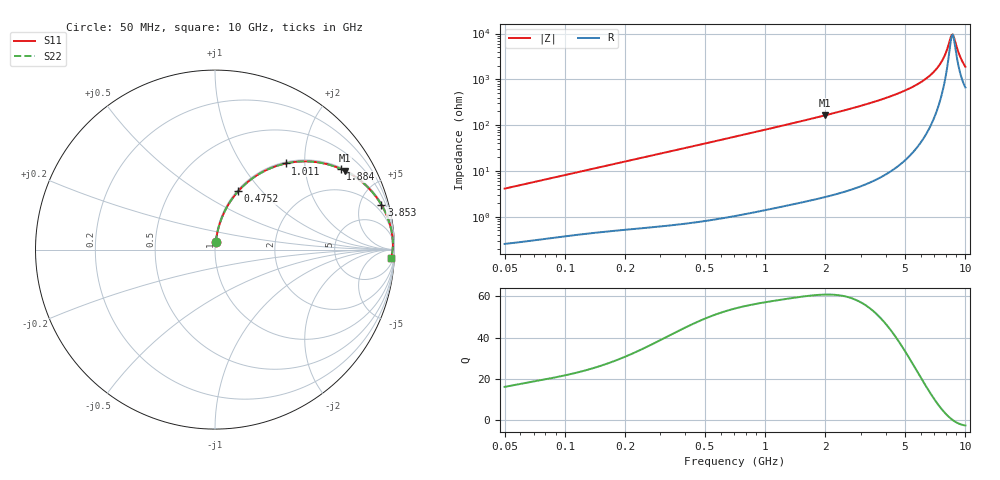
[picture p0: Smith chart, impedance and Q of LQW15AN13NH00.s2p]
!Murata Part Number: LQW15AN13NH00
!These Parameters are Measured in Series Mode Connection
!  o--[Z]--o
!Port1  Port2
!  o-------o
!Freq. Start=50[MHz] Stop=10[GHz], 401[Steps]
# Hz S RI R 50
!Freq.(Hz)	S 11(Real)	S 11(Imag)	S 21(Real)	S 21(Imag)	S 12(Real)	S 12(Imag)	S 22(Real)	S 22(Imag)
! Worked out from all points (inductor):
!   401 points, 50 MHz to 10 GHz, reference 50 ohm
!   read as one part in series: L = 13 nH near 51.34 MHz
!   highest Q = 60.9 at 1.987 GHz (marker M1), where L = 13 nH
!   self-resonance near 8.53 GHz
!   S11 on the Smith chart (normalised r, x): 50 MHz: 1.01, +0.08; 475.2 MHz: 1.02, +0.75; 1.011 GHz: 1.03, +1.60; 1.884 GHz: 1.05, +3.07; 3.853 GHz: 1.15, +7.37; 10 GHz: 14, -35
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5e7  0.00419 0.0406  0.9958 -0.0406  0.9958 -0.0406  0.00419 0.0406
1.214486e8  0.0134 0.0958  0.9866 -0.0958  0.9866 -0.0958  0.0134 0.0958
2.949953e8  0.0569 0.219  0.9431 -0.219  0.9431 -0.219  0.0569 0.219
4.752343e8  0.1287 0.3247  0.8713 -0.3247  0.8713 -0.3247  0.1287 0.3247
7.071068e8  0.2422 0.4193  0.7578 -0.4193  0.7578 -0.4193  0.2422 0.4193
1.011124e9  0.3935 0.4799  0.6065 -0.4799  0.6065 -0.4799  0.3935 0.4799
1.717543e9  0.6568 0.4666  0.3432 -0.4666  0.3432 -0.4666  0.6568 0.4666
1.884411e9  0.6996 0.4503  0.3004 -0.4503  0.3004 -0.4503  0.6996 0.4503
1.986945e9  0.7229 0.4394  0.2771 -0.4394  0.2771 -0.4394  0.7229 0.4394
2.766943e9  0.8458 0.3527  0.1542 -0.3527  0.1542 -0.3527  0.8458 0.3527
3.853138e9  0.927 0.2501  0.073 -0.2501  0.073 -0.2501  0.927 0.2501
4.171863e9  0.9408 0.225  0.0592 -0.225  0.0592 -0.225  0.9408 0.225
5.583245e9  0.9761 0.1344  0.0239 -0.1344  0.0239 -0.1344  0.9761 0.1344
6.810442e9  0.9882 0.0736  0.0118 -0.0736  0.0118 -0.0736  0.9882 0.0736
7.276762e9  0.9902 0.0534  0.00984 -0.0534  0.00984 -0.0534  0.9902 0.0534
7.672705e9  0.9909 0.037  0.00906 -0.037  0.00906 -0.037  0.9909 0.037
7.983737e9  0.991 0.0247  0.00899 -0.0247  0.00899 -0.0247  0.991 0.0247
8.418147e9  0.9903 0.00803  0.00967 -0.00803  0.00967 -0.00803  0.9903 0.00803
8.530394e9  0.99 0.00383  0.00999 -0.00383  0.00999 -0.00383  0.99 0.00383
8.759398e9  0.9892 -0.00462  0.0108 0.00462  0.0108 0.00462  0.9892 -0.00462
9.48396e9  0.9846 -0.0304  0.0154 0.0304  0.0154 0.0304  0.9846 -0.0304
1e10  0.9792 -0.048  0.0208 0.048  0.0208 0.048  0.9792 -0.048
